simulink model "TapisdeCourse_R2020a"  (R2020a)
settings: Solver=FixedStepAuto  StartTime=0.0  StopTime=30  FixedStep=1e-3  RelTol=1e-3  EnableMultiTasking=on
libraries: fl_lib x18, nesl_utility x11, fl_ps_legacy_lib x1, ee_lib x1

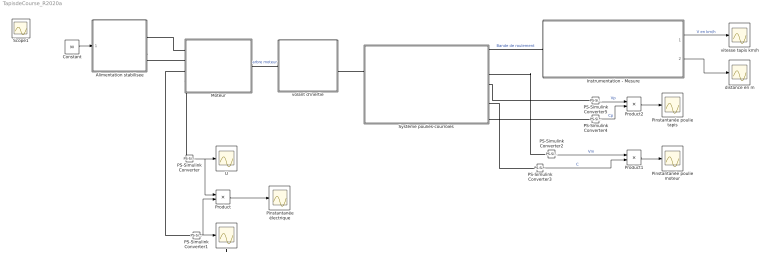
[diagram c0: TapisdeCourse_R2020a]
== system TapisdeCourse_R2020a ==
  Alimentation stabilisee : Subsystem
  Constant : Constant  Value=90
  I : Scope
  Instrumentation - Mesure : Subsystem
  Moteur : Subsystem  mask{R=1.7, L=1.2e-5, Kv=0.017, J=0.000971, Cs=0.076936, Cv=0.000159}
      mask prompts: R "Résistance R en Ohms"; L "Inductance de l'induit L en Henrys"; Kv "Constante de vitesse Kv en V/tr.min-1"; J "Moment d'inertie du Moteur J en Kg.m²"; Cs "Couple de frottements secs Cs en N.m"; Cv "Couple de frottements visqueux Cv en N.m/(rad/s)"
  PS-Simulink Converter{,1..5} (6 alike) : nesl_utility/PS-Simulink Converter  PhysicalDomain=network_engine_domain  SubClassName=ps_output  LeftPortType=input  RightPortType=output  PseudoPeriodic=off  Frequencies=[]  VectorFormat=1-D array  Unit=1  AffineConversion=off
  Pinstantanée poulie moteur : Scope
  Pinstantanée poulie tapis : Scope
  Pinstantanée électrique : Scope
  Product : Product
  Product1 : Product
  Product2 : Product
  Système poulies-courroies : Subsystem  mask{rapportreduction=3.3, rayonrouleau=20.75e-3}
      mask prompts: rapportreduction "Rapport de réduction du système poulies-courroie"; rayonrouleau "Rayon du rouleau entrainant r en m"
  U : Scope
  distance en m : Scope
  vitesse tapis km/h : Scope
  volant d'inertie : Subsystem  mask{inertie=0.007860}
      mask prompts: inertie "Inertie en kg.m²"
  Scope1 : Scope
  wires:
  PS-Simulink Converter/1 -> Product/1, U/1
  PS-Simulink Converter1/1 -> Product/2, I/1
  Product/1 -> Pinstantanée électrique/1
  PS-Simulink Converter2/1 -> Product1/1  "Vm"
  PS-Simulink Converter3/1 -> Product1/2  "C"
  Product1/1 -> Pinstantanée poulie moteur/1
  Constant/1 -> Alimentation stabilisee/1(In1)
  Product2/1 -> Pinstantanée poulie tapis/1
  PS-Simulink Converter5/1 -> Product2/1  "Vp"
  PS-Simulink Converter4/1 -> Product2/2  "Cp"
  Instrumentation - Mesure/1(Vitesse linéaire en km/h) -> vitesse tapis km/h/1  "V en km/h"
  Instrumentation - Mesure/2(Vitesse linéaire en km/h1) -> distance en m/1
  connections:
  Moteur/LConn1 -- Alimentation stabilisee/RConn1
  volant d'inertie/LConn1 -- Moteur/RConn1  "arbre moteur"
  Système poulies-courroies/RConn1 -- Instrumentation - Mesure/LConn1  "Bande de roulement"
  volant d'inertie/RConn1 -- Système poulies-courroies/LConn1
  Alimentation stabilisee/RConn2 -- Moteur/LConn2
  PS-Simulink Converter2/LConn1 -- Système poulies-courroies/RConn3
  Système poulies-courroies/RConn4 -- PS-Simulink Converter5/LConn1
  Moteur/LConn4 -- PS-Simulink Converter/LConn1
  PS-Simulink Converter1/LConn1 -- Moteur/LConn3
  Système poulies-courroies/RConn6 -- PS-Simulink Converter3/LConn1
  Système poulies-courroies/RConn7 -- PS-Simulink Converter4/LConn1

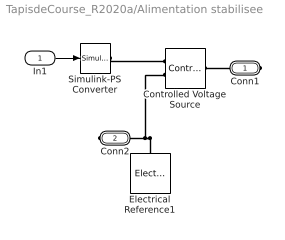
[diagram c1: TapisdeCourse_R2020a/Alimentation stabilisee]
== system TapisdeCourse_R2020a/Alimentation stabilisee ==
  In1 : Inport
  Controlled Voltage Source : fl_lib/Electrical/Electrical Sources/Controlled Voltage Source
  Electrical Reference1 : fl_lib/Electrical/Electrical Elements/Electrical Reference
  Simulink-PS Converter : nesl_utility/Simulink-PS Converter  PhysicalDomain=network_engine_domain  SubClassName=ps_input  LeftPortType=input  RightPortType=output  PseudoPeriodic=off  Frequencies=[]  NoiseDistribution=none  NoiseParameters=[]  Unit=1  AffineConversion=off  FilteringAndDerivatives=zero  SimscapeFilterOrder=1  InputFilterTimeConstant=.001  UdotUserProvided=0
  Conn1 : PMIOPort  Side=Right
  Conn2 : PMIOPort  Port=2  Side=Right
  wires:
  In1/1 -> Simulink-PS Converter/1
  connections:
  Simulink-PS Converter/RConn1 -- Controlled Voltage Source/RConn1
  Conn2/RConn1 -- Electrical Reference1/LConn1 -- Controlled Voltage Source/RConn2
  Conn1/RConn1 -- Controlled Voltage Source/LConn1

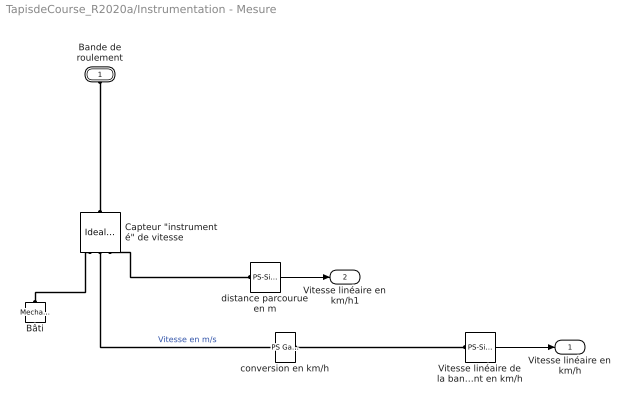
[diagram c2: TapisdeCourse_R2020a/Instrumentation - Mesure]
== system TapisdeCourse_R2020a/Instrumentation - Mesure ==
  Bâti : fl_lib/Mechanical/Translational Elements/Mechanical Translational Reference
  "Capteur \"instrumenté\" de vitesse" : fl_lib/Mechanical/Mechanical Sensors/Ideal Translational Motion Sensor  reference=foundation.enum.MeasurementReference.difference  acceleration_port=false  velocity_port=true  position_port=true  offset=0 m
  Vitesse linéaire de la bande de roulement en km/h : nesl_utility/PS-Simulink Converter  PhysicalDomain=network_engine_domain  SubClassName=ps_output  LeftPortType=input  RightPortType=output  PseudoPeriodic=off  Frequencies=[]  VectorFormat=1-D array  Unit=1  AffineConversion=off
  conversion en km/h : fl_ps_legacy_lib/Legacy Physical Signals/Functions/PS Gain  gain=3.6
  distance parcourue en m : nesl_utility/PS-Simulink Converter  PhysicalDomain=network_engine_domain  SubClassName=ps_output  LeftPortType=input  RightPortType=output  PseudoPeriodic=off  Frequencies=[]  VectorFormat=1-D array  Unit=1  AffineConversion=off
  Bande de roulement : PMIOPort  Side=Left
  Vitesse linéaire en km/h : Outport  VectorParamsAs1DForOutWhenUnconnected=off
  Vitesse linéaire en km/h1 : Outport  Port=2  VectorParamsAs1DForOutWhenUnconnected=off
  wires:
  Vitesse linéaire de la bande de roulement en km/h/1 -> Vitesse linéaire en km/h/1
  distance parcourue en m/1 -> Vitesse linéaire en km/h1/1
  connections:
  Bâti/LConn1 -- "Capteur \"instrumenté\" de vitesse"/RConn1
  conversion en km/h/RConn1 -- Vitesse linéaire de la bande de roulement en km/h/LConn1
  "Capteur \"instrumenté\" de vitesse"/RConn2 -- conversion en km/h/LConn1  "Vitesse en m/s"
  "Capteur \"instrumenté\" de vitesse"/LConn1 -- Bande de roulement/RConn1
  distance parcourue en m/LConn1 -- "Capteur \"instrumenté\" de vitesse"/RConn3

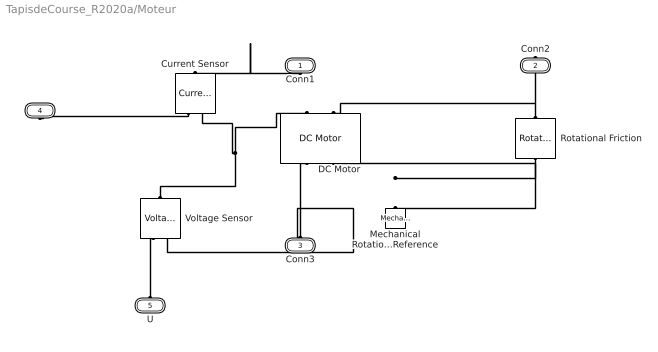
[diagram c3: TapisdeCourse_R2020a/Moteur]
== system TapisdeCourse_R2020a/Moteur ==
  Current Sensor : fl_lib/Electrical/Electrical Sensors/Current Sensor
  DC Motor : ee_lib/Electromechanical/Brushed Motors/DC Motor  field_option=ee.enum.field_option.pm  Rf=100 Ohm  Lf=1 H  Laf=0.15 H  If0=0 A  parameterization=1  Ra=R Ohm  La=L H  emf_or_torque=1  Kv=Kv V/rpm  Ki=6.876e-4 N*m/A  T_stall=2.4e-4 N*m  w_max=1.91e+4 rpm  w_rated=1.5e+4 rpm  P_rated=0.08 W  V_rated=1.5 V  lam_param=1  i_noload=0 A  V_i_noload=1.5 V  J=0.000971 kg*m^2  lam=0 N*m/(rad/s)  speed0=0 rpm  enable_fault_armature=simscape.enum.onoff.off  rev_faulted=1 / 3  G_faulted_armature=1e-5 S  fault_trigger_armature=ee.enum.faults.faultTrigger.temporal  t_fault_armature=1 s  max_permissible_current_armature=inf A  t_fail_on_current_armature=1 s  enable_fault_field=simscape.enum.onoff.off  G_faulted_field=1e-5 S  fault_trigger_field=ee.enum.faults.faultTrigger.temporal  t_fault_field=1 s  max_permissible_current_field=inf A  t_fail_on_current_field=1 s  fault_action=simscape.enum.assert.action.none  alpha=3.93e-3 1/K  Tmeas=25 degC  thermal_mass=100 J/K  initial_temperature=25 degC
  Mechanical Rotational Reference : fl_lib/Mechanical/Rotational Elements/Mechanical Rotational Reference
  Rotational Friction : fl_lib/Mechanical/Rotational Elements/Rotational Friction  brkwy_trq=Cs*1.25 N*m  brkwy_vel=0.60653 rad/s  Col_trq=Cs N*m  visc_coef=Cv N*m/(rad/s)  w_specify=off  w_priority=None  w=0 rad/s  w_nominal_specify=off  w_nominal_unit=rad/s  w_nominal_value=1  t_specify=off  t_priority=None  t=0 N*m  t_nominal_specify=off  t_nominal_unit=N*m  t_nominal_value=1
  Voltage Sensor : fl_lib/Electrical/Electrical Sensors/Voltage Sensor
  Conn1 : PMIOPort  Side=Left
  Conn2 : PMIOPort  Port=2  Side=Right
  Conn3 : PMIOPort  Port=3  Side=Left
  I : PMIOPort  Port=4  Side=Left
  U : PMIOPort  Port=5  Side=Left
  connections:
  Rotational Friction/LConn1 -- DC Motor/LConn2 -- Conn2/RConn1
  Conn3/RConn1 -- Voltage Sensor/RConn2 -- DC Motor/RConn1
  Rotational Friction/RConn1 -- DC Motor/RConn2 -- Mechanical Rotational Reference/LConn1
  Voltage Sensor/LConn1 -- Current Sensor/RConn2 -- DC Motor/LConn1
  Current Sensor/RConn1 -- I/RConn1
  U/RConn1 -- Voltage Sensor/RConn1
  Conn1/RConn1 -- Current Sensor/LConn1

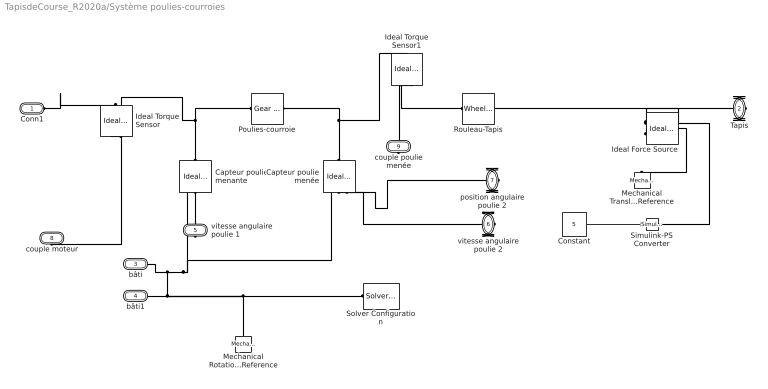
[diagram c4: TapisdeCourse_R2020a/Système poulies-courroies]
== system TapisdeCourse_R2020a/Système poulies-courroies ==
  Capteur poulie menée : fl_lib/Mechanical/Mechanical Sensors/Ideal Rotational Motion Sensor  reference=foundation.enum.MeasurementReference.difference  acceleration_port=false  velocity_port=true  position_port=true  wrap_angle=simscape.enum.onoff.off  offset=0 rad
  Capteur poulie menante : fl_lib/Mechanical/Mechanical Sensors/Ideal Rotational Motion Sensor  reference=foundation.enum.MeasurementReference.difference  acceleration_port=false  velocity_port=true  position_port=true  wrap_angle=simscape.enum.onoff.off  offset=0 rad
  Constant : Constant  Value=5
  Ideal Force Source : fl_lib/Mechanical/Mechanical Sources/Ideal Force Source
  Ideal Torque Sensor : fl_lib/Mechanical/Mechanical Sensors/Ideal Torque Sensor
  Ideal Torque Sensor1 : fl_lib/Mechanical/Mechanical Sensors/Ideal Torque Sensor
  Mechanical Rotational Reference : fl_lib/Mechanical/Rotational Elements/Mechanical Rotational Reference
  Mechanical Translational Reference : fl_lib/Mechanical/Translational Elements/Mechanical Translational Reference
  Poulies-courroie : fl_lib/Mechanical/Mechanisms/Gear Box  ratio=rapportreduction  t_in_specify=off  t_in_priority=None  t_in=0 N*m  t_in_nominal_specify=off  t_in_nominal_unit=N*m  t_in_nominal_value=1  t_out_specify=off  t_out_priority=None  t_out=0 N*m  t_out_nominal_specify=off  t_out_nominal_unit=N*m  t_out_nominal_value=1
  Rouleau-Tapis : fl_lib/Mechanical/Mechanisms/Wheel and Axle  R=rayonrouleau m  or=1  t_specify=off  t_priority=None  t=0 N*m  t_nominal_specify=off  t_nominal_unit=N*m  t_nominal_value=1  f_specify=off  f_priority=None  f=0 N  f_nominal_specify=off  f_nominal_unit=N  f_nominal_value=1
  Simulink-PS Converter : nesl_utility/Simulink-PS Converter  PhysicalDomain=network_engine_domain  SubClassName=ps_input  LeftPortType=input  RightPortType=output  PseudoPeriodic=off  Frequencies=[]  NoiseDistribution=none  NoiseParameters=[]  Unit=1  AffineConversion=off  FilteringAndDerivatives=provide  SimscapeFilterOrder=1  InputFilterTimeConstant=0.001  UdotUserProvided=0
  Solver Configuration : nesl_utility/Solver Configuration  PhysicalDomain=network_engine_domain  SubClassName=solver  LeftPortType=input  RightPortType=generic  Tones=[]  Harmonics=[]  SimulateNoise=off  Profile=off  UseLocalSampling=off  EnableSwitchedLinearOptims=on  FrequencyDomain=off  UseCCode=off  RelTol=0.001  AbsTol=1e-06  MinStep=1e-09  ToWorkspace=off  RevertToSquareIcSolve=off  NumHomotopyIterations=100  PhasorMode=off  PhasorModeNumHarmonics=1  ConsistencySolver=NEWTON_FTOL  IndexReductionMethod=DerivativeReplacement  DoDC=on  ResidualTolerance=1e-9  ConsistencyTolSource=GLOBAL  ConsistencyAbsTol=0.001  ConsistencyRelTol=0.001  ConsistencyTolFactor=0.001  UseLocalSolver=off  LocalSolverChoice=NE_BACKWARD_EULER_ADVANCER  ResolveIndetEquations=on  FunctionEvalNumThread=1  LocalSolverSampleTime=.001  DoFixedCost=off  MaxNonlinIter=3  MaxModeIter=2  ComputeImpulses=off  ImpulseIterations=2  LinearAlgebra=Sparse  LinearAlgebraNumThread=0  EquationFormulation=NE_TIME_EF  DelaysMemoryBudget=1024  AutomaticFiltering=on  FilteringTimeConstant=0.001  PartitionStorageMethod=AS_NEEDED  PartitionMemoryBudget=1024  PartitionMethod=FAST  MultibodyUseLocalSolver=off  MultibodyLocalSolverChoice=ODE1  MultibodyLocalSolverSampleTime=0.001
  Conn1 : PMIOPort  Side=Left
  Tapis : PMIOPort  Port=2  Side=Right
  bâti : PMIOPort  Port=3  Side=Left
  bâti1 : PMIOPort  Port=4  Side=Right
  vitesse angulaire poulie 1 : PMIOPort  Port=5  Side=Right
  vitesse angulaire poulie 2 : PMIOPort  Port=6  Side=Right
  position angulaire poulie 2 : PMIOPort  Port=7  Side=Right
  couple moteur : PMIOPort  Port=8  Side=Right
  couple poulie menée : PMIOPort  Port=9  Side=Right
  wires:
  Constant/1 -> Simulink-PS Converter/1
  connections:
  Capteur poulie menante/LConn1 -- Poulies-courroie/LConn1 -- Ideal Torque Sensor/RConn1
  Capteur poulie menée/LConn1 -- Ideal Torque Sensor1/LConn1 -- Poulies-courroie/RConn1
  vitesse angulaire poulie 1/RConn1 -- Capteur poulie menante/RConn2
  Mechanical Rotational Reference/LConn1 -- Solver Configuration/RConn1 -- bâti/RConn1 -- Capteur poulie menante/RConn1 -- Capteur poulie menée/RConn1 -- bâti1/RConn1
  vitesse angulaire poulie 2/RConn1 -- Capteur poulie menée/RConn2
  position angulaire poulie 2/RConn1 -- Capteur poulie menée/RConn3
  Ideal Torque Sensor/RConn2 -- couple moteur/RConn1
  Conn1/RConn1 -- Ideal Torque Sensor/LConn1
  Ideal Force Source/RConn2 -- Rouleau-Tapis/RConn1 -- Tapis/RConn1
  Simulink-PS Converter/RConn1 -- Ideal Force Source/RConn1
  Ideal Force Source/LConn1 -- Mechanical Translational Reference/LConn1
  Ideal Torque Sensor1/RConn1 -- Rouleau-Tapis/LConn1
  couple poulie menée/RConn1 -- Ideal Torque Sensor1/RConn2

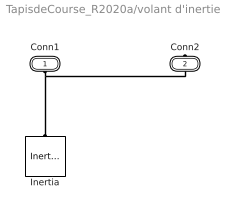
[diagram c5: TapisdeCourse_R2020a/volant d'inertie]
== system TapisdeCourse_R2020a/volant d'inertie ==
  Inertia : fl_lib/Mechanical/Rotational Elements/Inertia  inertia=inertie kg*m^2  num_ports=foundation.enum.numPorts2.one  w_specify=on  w_priority=High  w=0 rad/s  w_nominal_specify=off  w_nominal_unit=rad/s  w_nominal_value=1  t_specify=off  t_priority=None  t=0 N*m  t_nominal_specify=off  t_nominal_unit=N*m  t_nominal_value=1
  Conn1 : PMIOPort  Side=Left
  Conn2 : PMIOPort  Port=2  Side=Right
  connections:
  Conn1/RConn1 -- Conn2/RConn1 -- Inertia/LConn1
